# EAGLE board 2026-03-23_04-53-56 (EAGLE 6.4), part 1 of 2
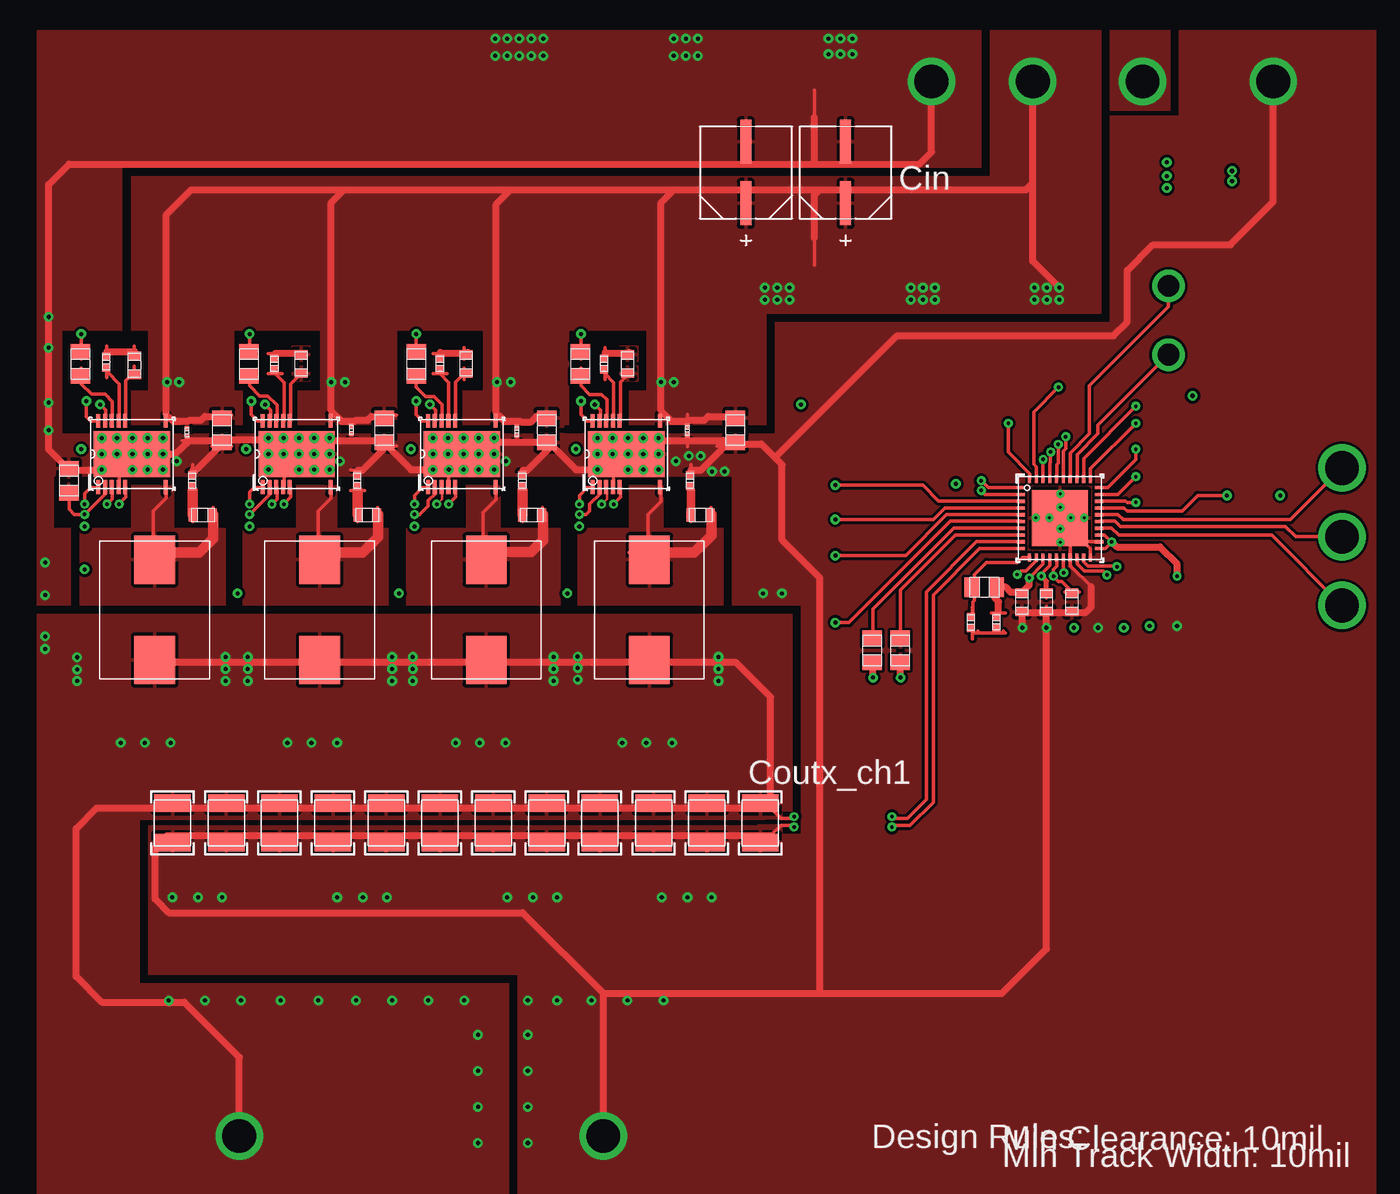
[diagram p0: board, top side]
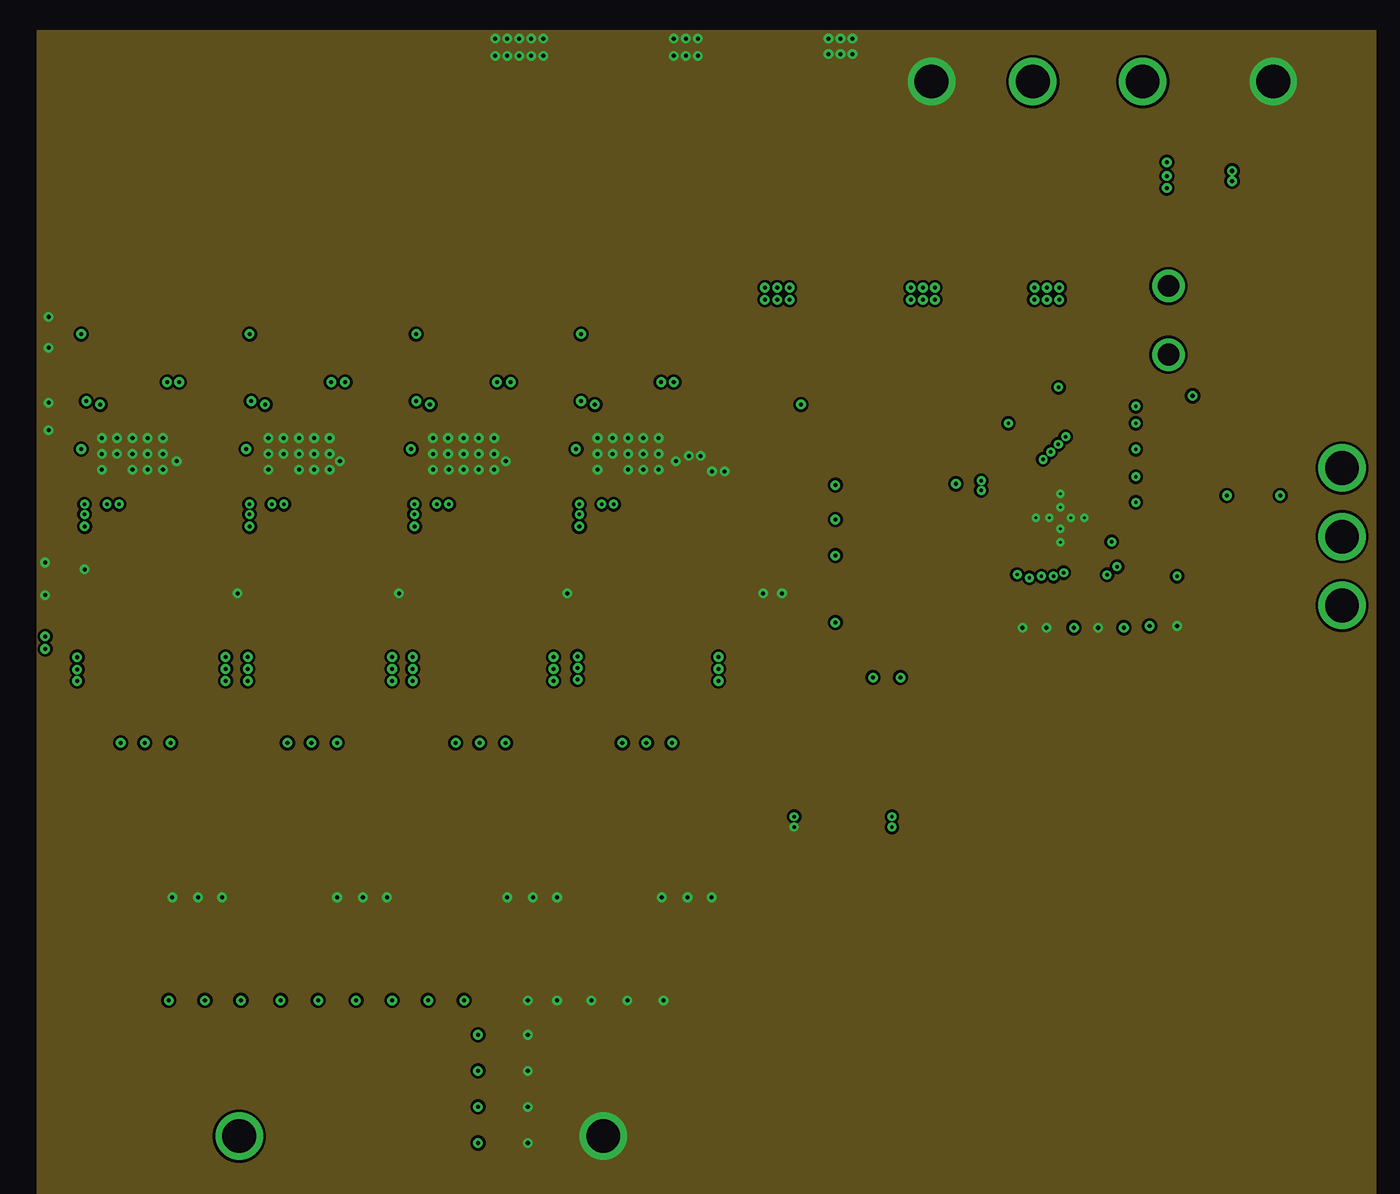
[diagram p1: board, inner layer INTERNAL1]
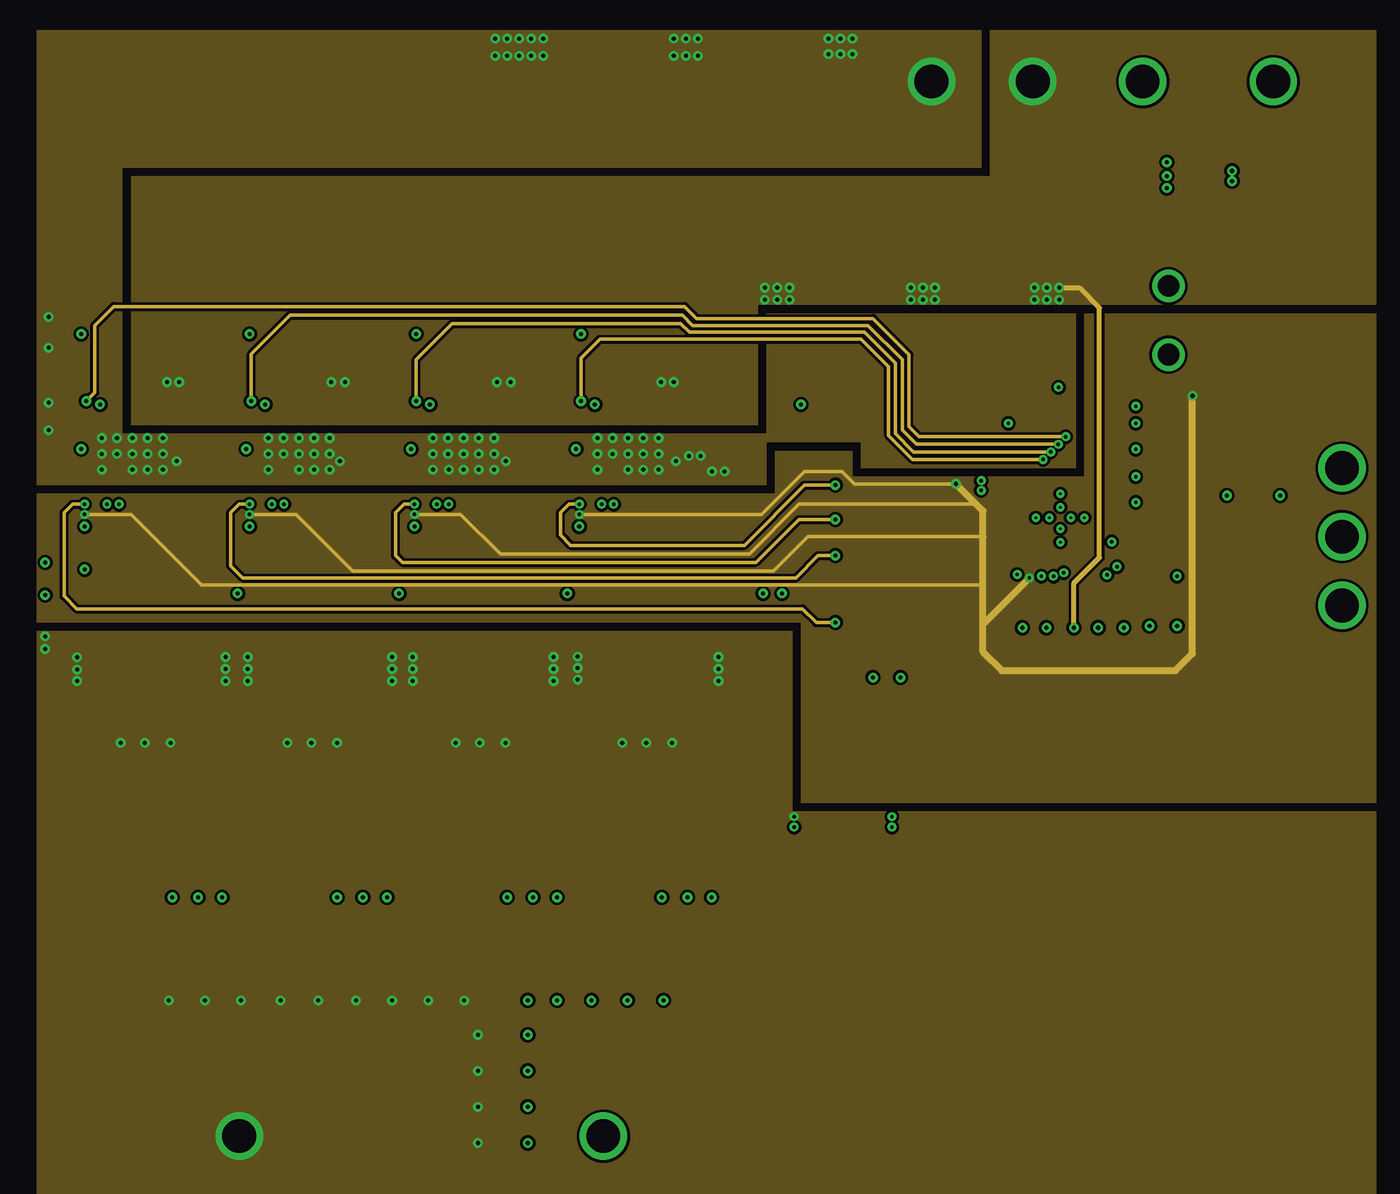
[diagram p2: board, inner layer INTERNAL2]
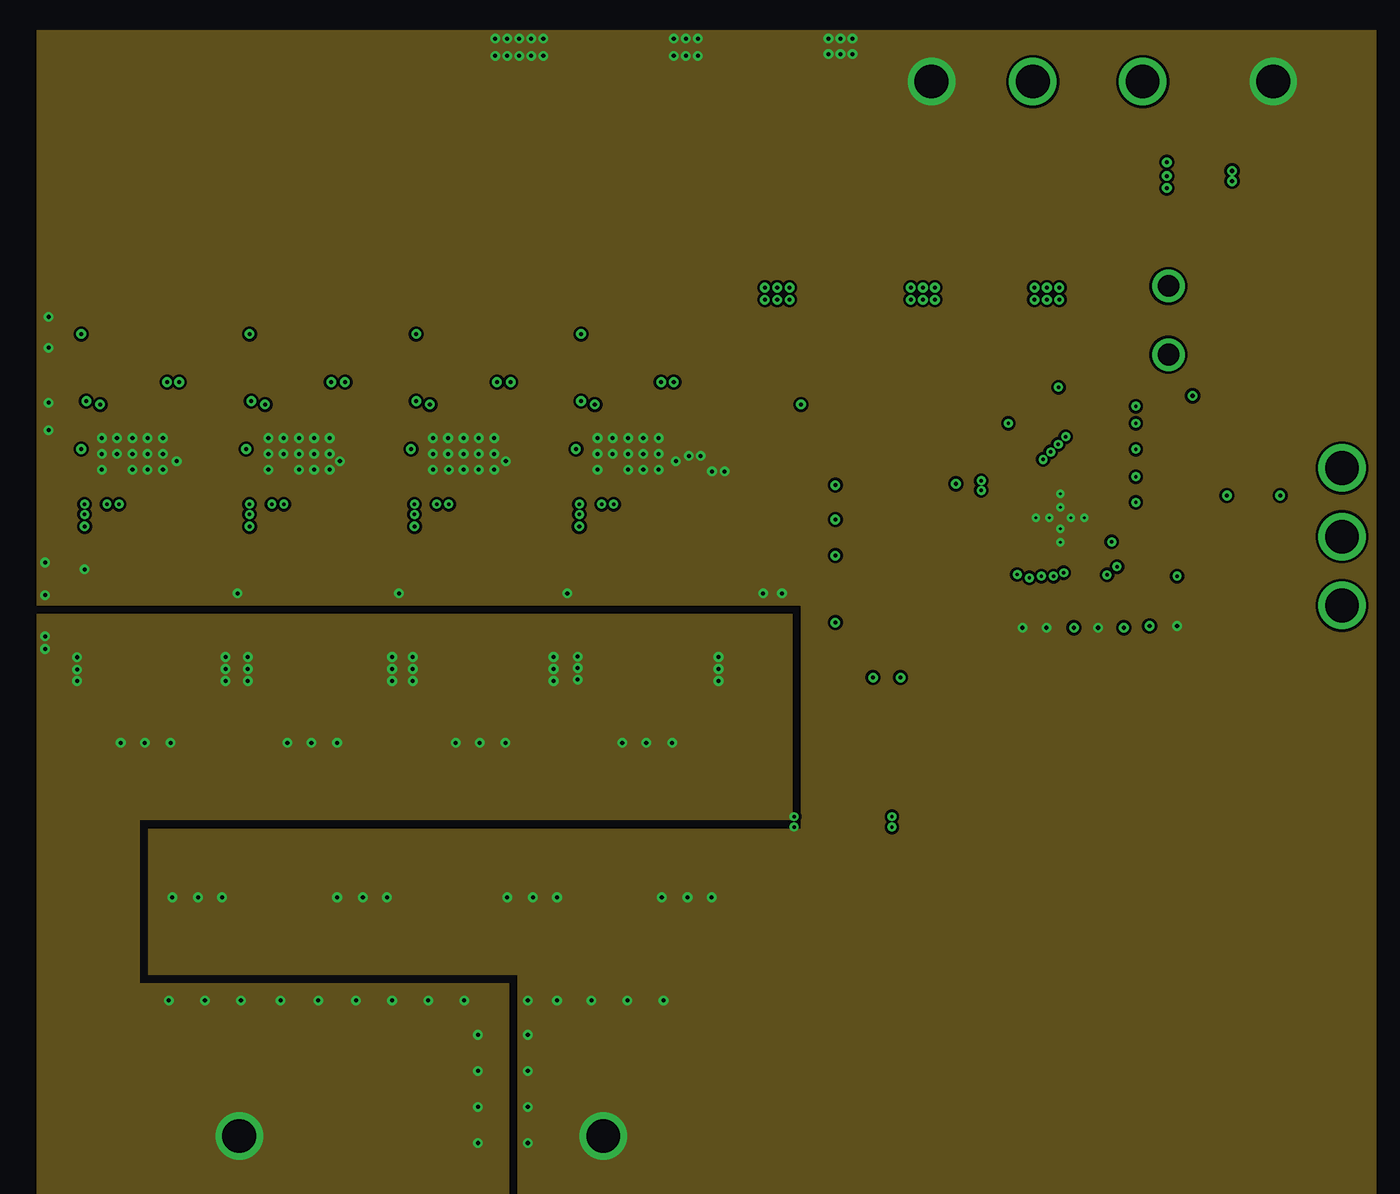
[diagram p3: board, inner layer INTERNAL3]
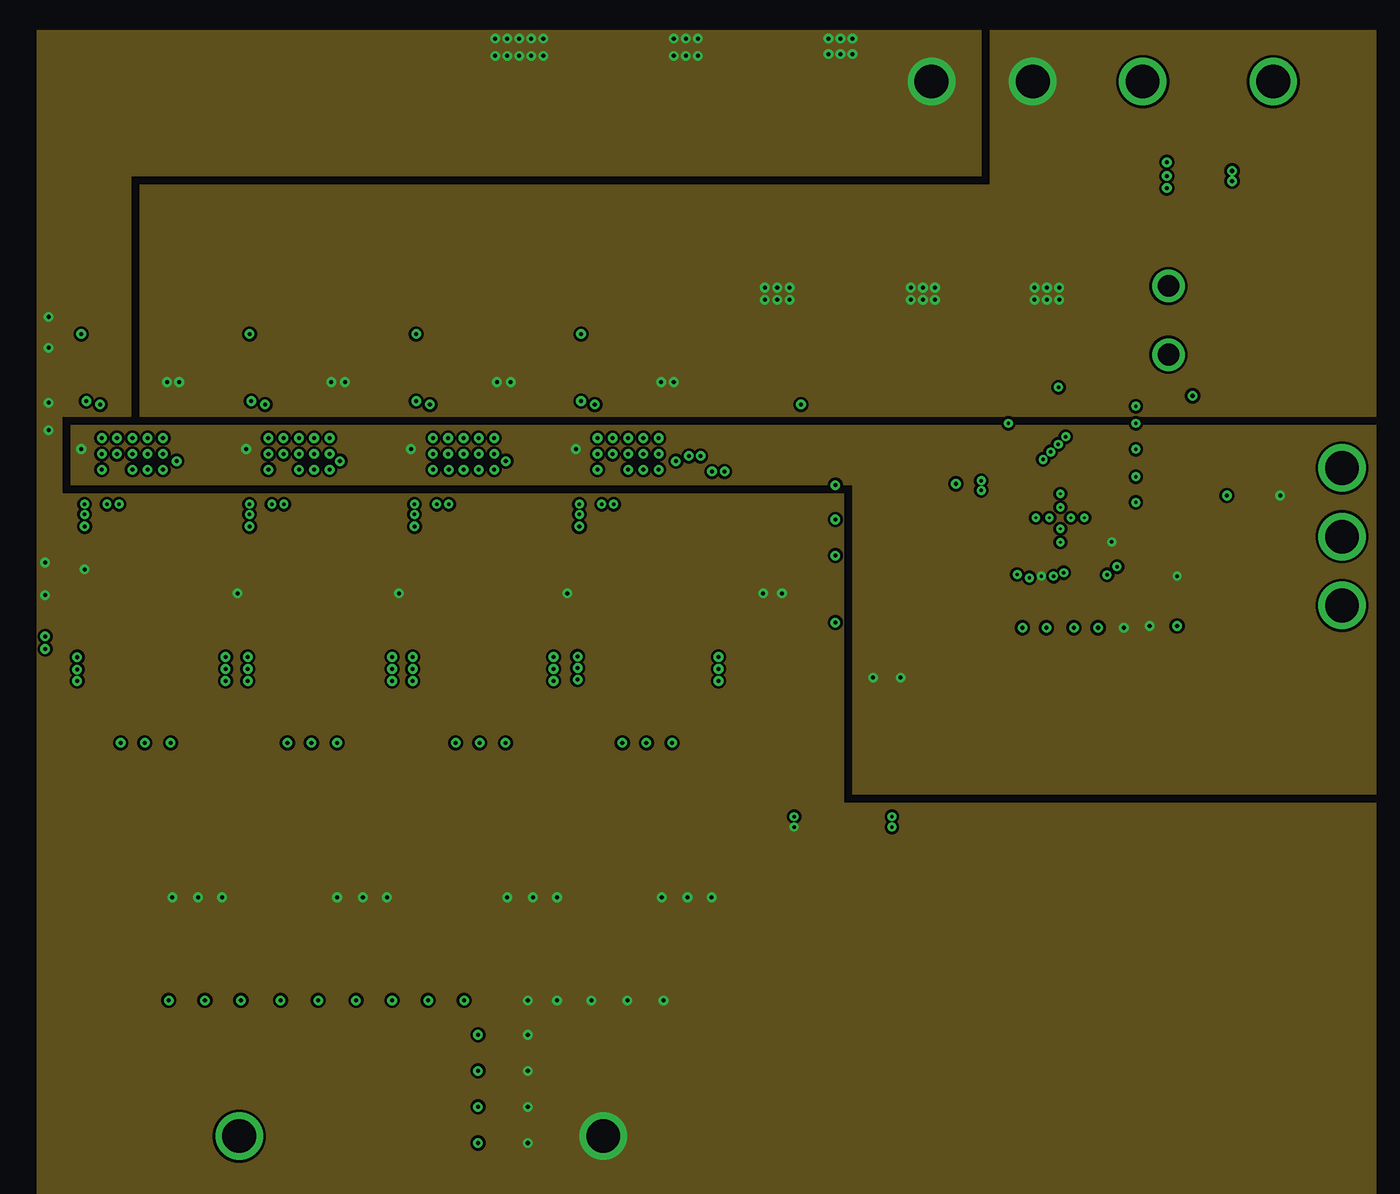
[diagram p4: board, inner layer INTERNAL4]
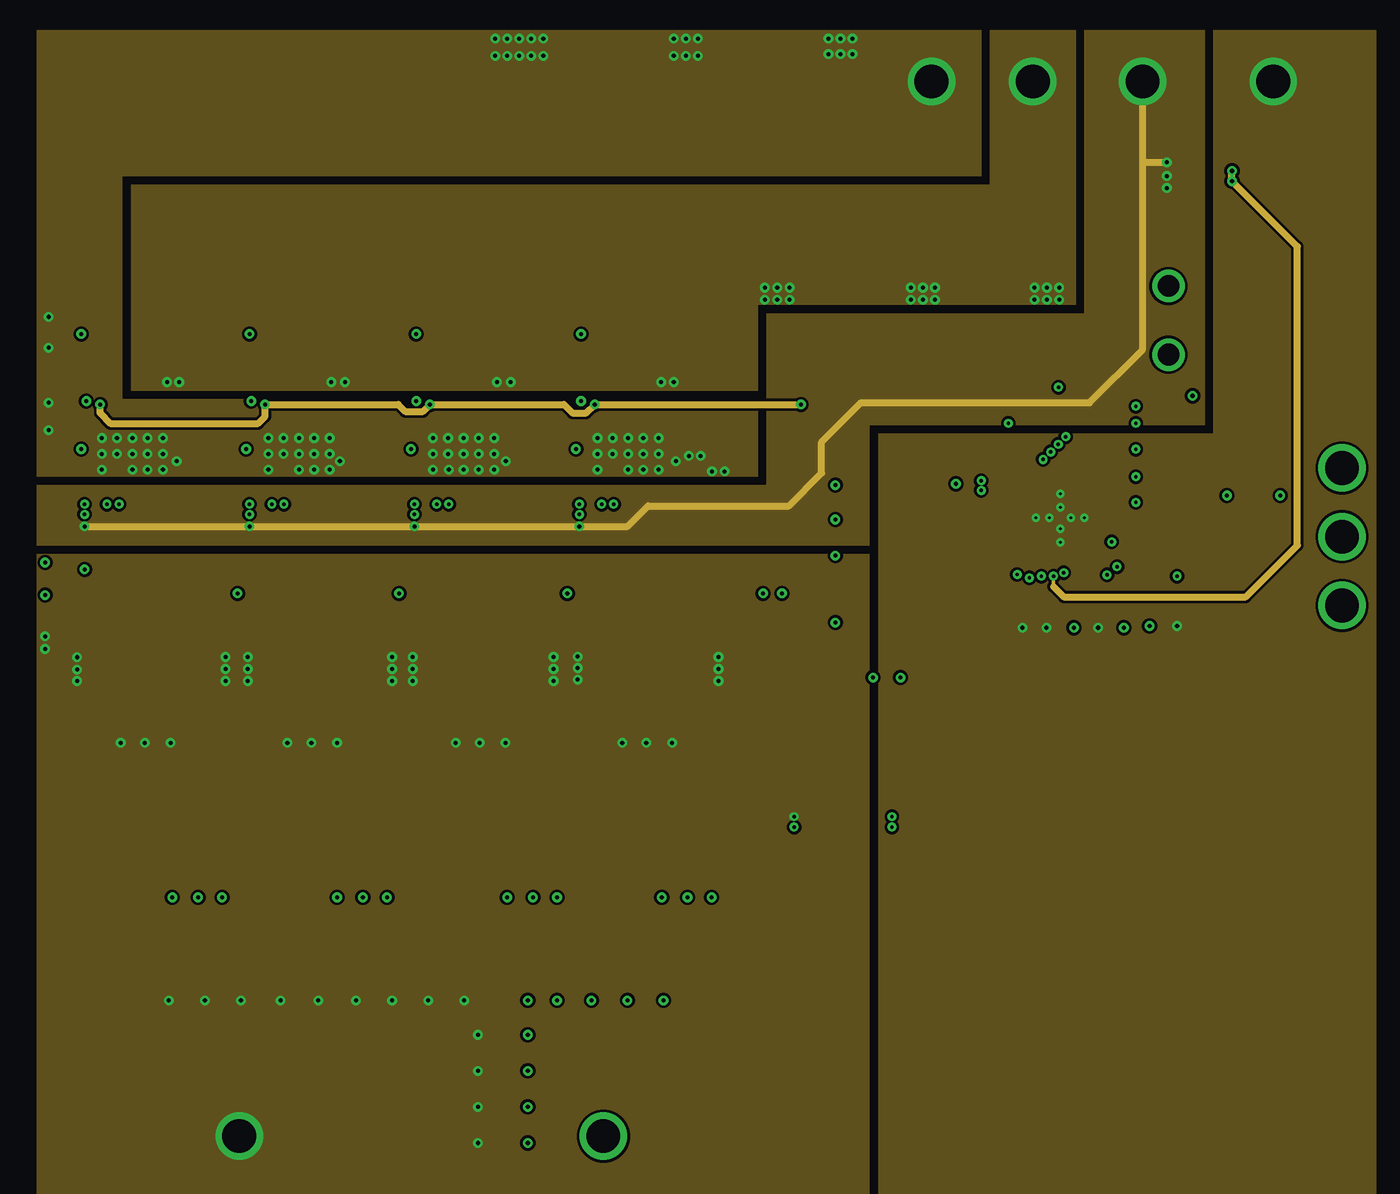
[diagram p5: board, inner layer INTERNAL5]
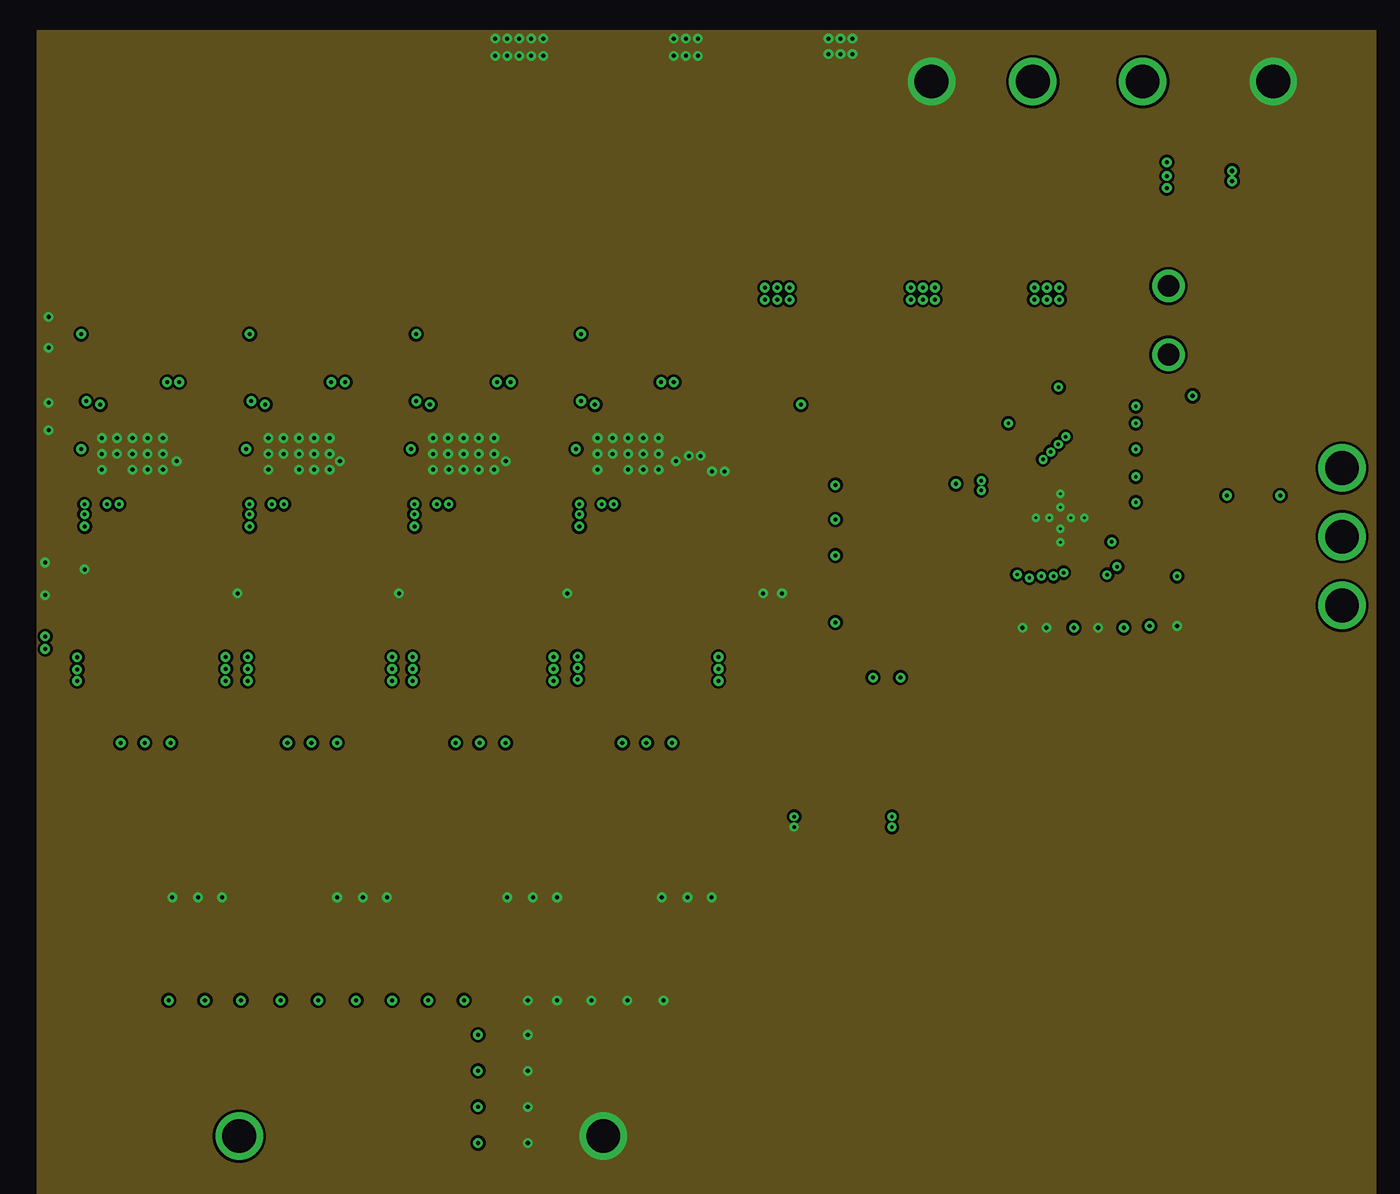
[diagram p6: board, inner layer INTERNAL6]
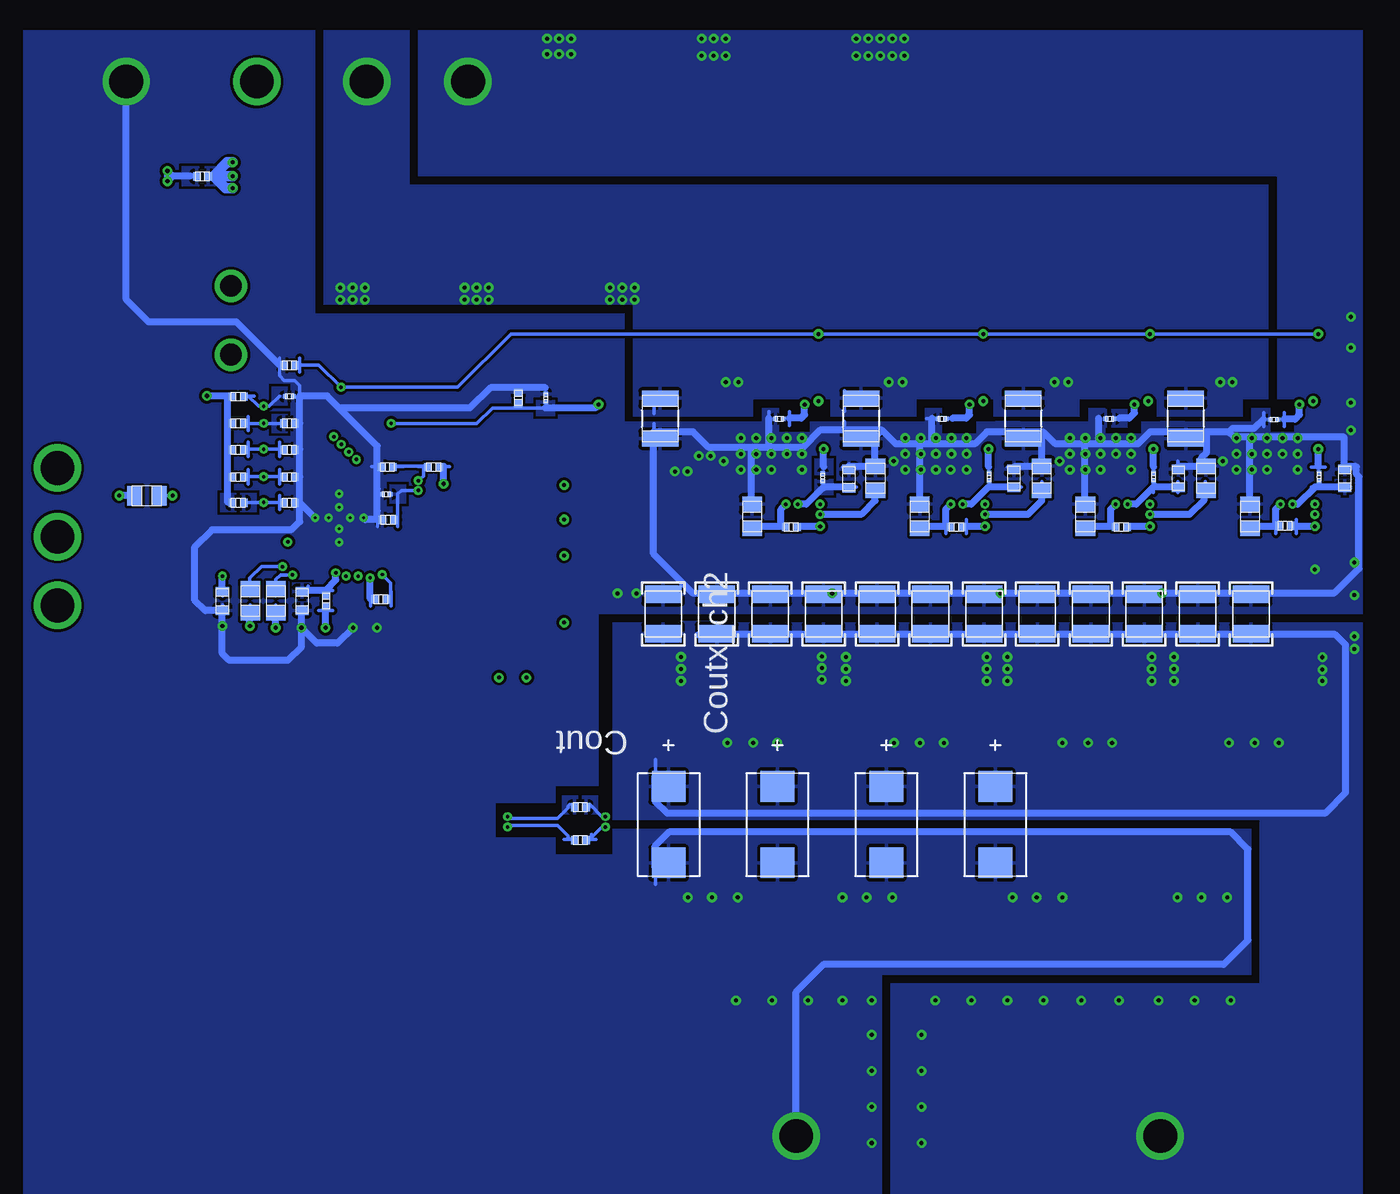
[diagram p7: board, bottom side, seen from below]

No outline drawn. Coordinates in mm, seen from the top.
Copper layers ((1*2)+(15*16)): TOP / INTERNAL1 / layer 15 / BOTTOM

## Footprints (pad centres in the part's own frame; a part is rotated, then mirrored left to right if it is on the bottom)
0603 = smd 0.66 x 0.965: 1 -0.699,0; 2 0.699,0
0402 = smd 0.559 x 0.61: 1 -0.419,0; 2 0.419,0
0805 = smd 1.118 x 1.448: 1 -0.902,0; 2 0.902,0
0201_033 = smd 0.356 x 0.33: 1 -0.292,0; 2 0.292,0
0201 = smd 0.356 x 0.33: 1 -0.292,0; 2 0.292,0
CAPSMT_62_C10 = smd 3.251 x 0.813: 1 -2.273,0; 2 2.273,0
1210_280 = smd 1.118 x 2.692: 1 -1.499,0; 2 1.499,0
7343-20 = smd 2.261 x 2.489: 1 -2.819,0; 2 2.819,0
1210_270 = smd 1.3 x 2.7: 1 -1.45,0; 2 1.45,0
TP-1502 = drill 0.813 pad 1.651 round: 1 0,0
WE-HCM_1088 = smd 3.56 x 3: 1 -3.71,0; 2 3.71,0
DQP0012A = smd 1 x 0.3: 1 -2.45,2.501; 2 -2.45,2.001; 3 -2.45,1.5; 4 -2.45,1; 5 -2.45,0.5; 6 -2.45,-2.501; 7 2.45,-2.501; 8 2.45,0.5; 9 2.45,1; 10 2.45,1.5; 11 2.45,2.001; 12 2.45,2.501 | smd 3.4 x 5.639: 13 0,0
TP-5012 = drill 0.813 pad 1.651 round: 1 0,0
RTA0040B = smd 0.6 x 0.23: 1 -2.9,2.25; 2 -2.9,1.75; 3 -2.9,1.25; 4 -2.9,0.75; 5 -2.9,0.25; 6 -2.9,-0.25; 7 -2.9,-0.75; 8 -2.9,-1.25; 9 -2.9,-1.75; 10 -2.9,-2.25; 21 2.9,-2.25; 22 2.9,-1.75; 23 2.9,-1.25; 24 2.9,-0.75; 25 2.9,-0.25; 26 2.9,0.25; 27 2.9,0.75; 28 2.9,1.25; 29 2.9,1.75; 30 2.9,2.25 | smd 0.23 x 0.6: 11 -2.25,-2.9; 12 -1.75,-2.9; 13 -1.25,-2.9; 14 -0.75,-2.9; 15 -0.25,-2.9; 16 0.25,-2.9; 17 0.75,-2.9; 18 1.25,-2.9; 19 1.75,-2.9; 20 2.25,-2.9; 31 2.25,2.9; 32 1.75,2.9; 33 1.25,2.9; 34 0.75,2.9; 35 0.25,2.9; 36 -0.25,2.9; 37 -0.75,2.9; 38 -1.25,2.9; 39 -1.75,2.9; 40 -2.25,2.9 | smd 4.15 x 4.15: 41 0,0

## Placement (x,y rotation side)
C3v3  [0603]  111,70.82 270 bottom
Cbp3  [0603]  101.35,70.71 270 top
Cbst1  [0603]  70.36,88.34 270 top
Cbst2  [0603]  58.42,88.34 270 top
Cbst3  [0603]  46.23,88.34 270 top
Cbst4  [0603]  33.91,88.24 270 top
Ccomp  [0402]  97.64,69.24 90 top
Ccomp2  [0805]  96.75,71.83 0 top
Cdd  [0603]  105.11,70.82 270 bottom
Cen1  [0603]  64.67,79.86 90 bottom
Cen2  [0603]  52.48,79.88 90 bottom
Cen3  [0603]  40.31,79.88 90 bottom
Cen4  [0603]  28.02,79.88 90 bottom
Chf1  [0201_033]  74.78,83.41 270 top
Chf2  [0201_033]  62.18,83.34 270 top
Chf3  [0201_033]  49.96,83.46 270 top
Chf4  [0201_033]  37.8,83.29 270 top
Cimon  [0201]  98.88,78.71 180 bottom
Cin_1  [CAPSMT_62_C10]  86.49,102.49 90 top
Cin_2  [CAPSMT_62_C10]  79.12,102.49 90 top
Cinx_ch1  [0805]  78.33,83.44 270 top
Cinx_ch2  [0805]  64.39,83.44 270 top
Cinx_ch3  [0805]  52.37,83.44 270 top
Cinx_ch4  [0805]  40.39,83.44 270 top
Cinx_ch5  [1210_280]  78.64,84.3 270 bottom
Cinx_ch6  [1210_280]  63.78,84.3 270 bottom
Cinx_ch7  [1210_280]  51.79,84.3 270 bottom
Cinx_ch8  [1210_280]  39.78,84.3 270 bottom
Cout_1  [7343-20]  78,54.28 270 bottom
Cout_2  [7343-20]  69.95,54.28 270 bottom
Cout_3  [7343-20]  61.9,54.28 270 bottom
Cout_4  [7343-20]  53.85,54.28 270 bottom
Coutx_ch1_1  [1210_270]  80.19,54.41 270 top
Coutx_ch1_2  [1210_270]  76.23,54.41 270 top
Coutx_ch1_3  [1210_270]  72.29,54.41 270 top
Coutx_ch1_4  [1210_270]  68.33,54.41 270 top
Coutx_ch1_5  [1210_270]  64.39,54.41 270 top
Coutx_ch1_6  [1210_270]  60.43,54.41 270 top
Coutx_ch1_7  [1210_270]  56.49,54.41 270 top
Coutx_ch1_8  [1210_270]  52.53,54.41 270 top
Coutx_ch1_9  [1210_270]  48.59,54.41 270 top
Coutx_ch1_10  [1210_270]  44.63,54.41 270 top
Coutx_ch1_11  [1210_270]  40.69,54.41 270 top
Coutx_ch1_12  [1210_270]  36.73,54.41 270 top
Coutx_ch2_1  [1210_270]  78.41,69.85 90 bottom
Coutx_ch2_2  [1210_270]  74.45,69.85 90 bottom
Coutx_ch2_3  [1210_270]  70.48,69.85 90 bottom
Coutx_ch2_4  [1210_270]  66.55,69.85 90 bottom
Coutx_ch2_5  [1210_270]  62.59,69.85 90 bottom
Coutx_ch2_6  [1210_270]  58.65,69.85 90 bottom
Coutx_ch2_7  [1210_270]  54.69,69.85 90 bottom
Coutx_ch2_8  [1210_270]  50.75,69.85 90 bottom
Coutx_ch2_9  [1210_270]  46.79,69.85 90 bottom
Coutx_ch2_10  [1210_270]  42.85,69.85 90 bottom
Coutx_ch2_11  [1210_270]  38.89,69.85 90 bottom
Coutx_ch2_12  [1210_270]  34.95,69.85 90 bottom
Cref  [0603]  99.52,70.71 270 top
Cref1  [0805]  62.71,79.88 90 bottom
Cref2  [0805]  50.42,79.88 90 bottom
Cref3  [0805]  38.28,79.88 90 bottom
Cref4  [0805]  29.06,79.71 90 top
Csnub1  [0603]  75.77,77.17 180 top
Csnub2  [0603]  63.3,77.17 180 top
Csnub3  [0603]  51.13,77.17 180 top
Csnub4  [0603]  38.96,77.17 180 top
Ctao1  [0201]  69.82,84.28 180 bottom
Ctao2  [0201]  57.78,84.28 180 bottom
Ctao3  [0201]  45.39,84.28 180 bottom
Ctao4  [0201]  33.25,84.23 180 bottom
Ctsen  [0201]  87.07,85.83 90 bottom
Cv5  [0603]  103.23,70.71 270 top
Cvdd1  [0805]  71.83,77.06 90 bottom
Cvdd2  [0805]  59.44,77.06 90 bottom
Cvdd3  [0805]  47.19,77.06 90 bottom
Cvdd4  [0805]  35.03,77.06 90 bottom
GND  [TP-1502]  92.84,109.17 0 top
GND1  [TP-1502]  68.53,31.19 0 top
GND2  [TP-1502]  118.08,109.17 0 top
L1  [WE-HCM_1088]  71.98,70.15 270 top
L2  [WE-HCM_1088]  59.92,70.15 270 top
L3  [WE-HCM_1088]  47.6,70.15 270 top
L4  [WE-HCM_1088]  35.41,70.15 270 top
M1  [DQP0012A]  70.28,81.69 90 top
M2  [DQP0012A]  58.12,81.69 90 top
M3  [DQP0012A]  45.9,81.69 90 top
M4  [DQP0012A]  33.73,81.69 90 top
NC3  [TP-5012]  110.34,88.98 0 top
NC4  [TP-5012]  110.34,94.03 0 top
Raddr  [0402]  109.83,78.08 0 bottom
Rbst1  [0402]  68.63,88.34 270 top
Rbst2  [0402]  56.49,88.34 270 top
Rbst3  [0402]  44.25,88.34 270 top
Rbst4  [0402]  31.83,88.47 270 top
Rcomp  [0402]  95.76,69.22 90 top
Rdd  [0402]  103.33,70.82 270 bottom
Ren1  [0201]  66.6,79.93 270 bottom
Ren2  [0201]  54.31,79.98 270 bottom
Ren3  [0201]  42.14,79.98 270 bottom
Ren4  [0201]  29.92,79.98 270 bottom
Rf  [0201]  106.05,85.93 0 bottom
Rfccm1  [0805]  66.88,88.34 270 top
Rfccm2  [0805]  54.74,88.34 270 top
Rfccm3  [0805]  42.37,88.34 270 top
Rfccm4  [0805]  29.92,88.34 270 top
Rimax  [0402]  109.83,85.93 0 bottom
Rimon  [0402]  98.76,76.81 180 bottom
Risum  [0402]  99.29,70.94 0 bottom
Rmode  [0402]  109.83,79.98 0 bottom
Rnc1  [0805]  90.53,67.16 90 top
Rnc2  [0805]  88.47,67.16 90 top
Rnvm  [0402]  106.05,88.24 180 bottom
Rocpr  [0402]  98.81,80.72 180 bottom
Rosr  [0402]  106.05,81.99 0 bottom
Rramp  [0402]  95.38,80.72 180 bottom
Rslew  [0402]  106.05,79.98 0 bottom
Rsn  [0402]  84.53,53.14 180 bottom
Rsnub1  [0402]  74.98,79.71 90 top
Rsnub2  [0402]  62.59,79.71 90 top
Rsnub3  [0402]  50.37,79.71 90 top
Rsnub4  [0402]  38.18,79.71 90 top
Rsp  [0402]  84.53,55.58 180 bottom
Rtrise  [0402]  106.05,78.08 0 bottom
Rtsen  [0402]  89.13,85.83 90 bottom
Rusr  [0402]  109.83,81.99 0 bottom
Rv5  [0402]  112.47,102.21 180 bottom
Rvbootb  [0402]  106.05,83.95 0 bottom
Rvboott  [0402]  109.83,83.95 0 bottom
Rvdd1  [0402]  68.94,76.28 0 bottom
Rvdd2  [0402]  56.72,76.28 0 bottom
Rvdd3  [0402]  44.53,76.28 0 bottom
Rvdd4  [0402]  32.44,76.38 0 bottom
Rvr_fault  [0805]  116.59,78.59 0 bottom
Rvr_hot  [0805]  108.92,70.82 90 bottom
Rvr_rdy  [0805]  107.04,70.82 90 bottom
U1  [RTA0040B]  102.34,76.94 0 top
V5  [TP-1502]  108.43,109.17 0 top
Valert  [TP-1502]  123.16,75.54 0 top
VIN  [TP-1502]  100.28,109.17 0 top
VOUT  [TP-1502]  41.61,31.19 0 top
Vscl  [TP-1502]  123.16,70.48 0 top
Vsda  [TP-1502]  123.16,80.64 0 top

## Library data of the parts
C3v3 = ultra-librarian; RefDes: C3v3; Type: C0603C105Z8VACTU
Cbp3 = ultra-librarian; RefDes: Cbp3; Type: C0603C105Z8VACTU
Cbst1 = ultra-librarian; RefDes: Cbst1; Type: EMK107B7104KA-T
Cbst2 = ultra-librarian; RefDes: Cbst2; Type: EMK107B7104KA-T
Cbst3 = ultra-librarian; RefDes: Cbst3; Type: EMK107B7104KA-T
Cbst4 = ultra-librarian; RefDes: Cbst4; Type: EMK107B7104KA-T
Ccomp = ultra-librarian; RefDes: Ccomp; Type: GRM1555C1H102JA01J
Ccomp2 = ultra-librarian; RefDes: Ccomp2; Type: CL21C220JBANNNC
Cdd = ultra-librarian; RefDes: Cdd; Type: C1608X5R1E105K080AC
Cen1 = ultra-librarian; RefDes: Cen1; Type: CC0603JRNPO8BN102
Cen2 = ultra-librarian; RefDes: Cen2; Type: CC0603JRNPO8BN102
Cen3 = ultra-librarian; RefDes: Cen3; Type: CC0603JRNPO8BN102
Cen4 = ultra-librarian; RefDes: Cen4; Type: CC0603JRNPO8BN102
Chf1 = ultra-librarian; RefDes: Chf1; Type: CGA1A2X7R1E332K030BA
Chf2 = ultra-librarian; RefDes: Chf2; Type: CGA1A2X7R1E332K030BA
Chf3 = ultra-librarian; RefDes: Chf3; Type: CGA1A2X7R1E332K030BA
Chf4 = ultra-librarian; RefDes: Chf4; Type: CGA1A2X7R1E332K030BA
Cimon = ultra-librarian; RefDes: Cimon; Type: GRM033R71A222KA01D
Cin_1 Cin_2 Cout_1-Cout_4 Coutx_ch1_1-Coutx_ch1_12 Coutx_ch2_1-Coutx_ch2_12 M1-M4 = ultra-librarian
Cinx_ch1 = ultra-librarian; RefDes: Cinx_ch1; Type: MSASE21GBB5226MTNA01
Cinx_ch2 = ultra-librarian; RefDes: Cinx_ch2; Type: MSASE21GBB5226MTNA01
Cinx_ch3 = ultra-librarian; RefDes: Cinx_ch3; Type: MSASE21GBB5226MTNA01
Cinx_ch4 = ultra-librarian; RefDes: Cinx_ch4; Type: MSASE21GBB5226MTNA01
Cinx_ch5 = ultra-librarian; RefDes: Cinx_ch5; Type: GRM32ER61C476KE15L
Cinx_ch6 = ultra-librarian; RefDes: Cinx_ch6; Type: GRM32ER61C476KE15L
Cinx_ch7 = ultra-librarian; RefDes: Cinx_ch7; Type: GRM32ER61C476KE15L
Cinx_ch8 = ultra-librarian; RefDes: Cinx_ch8; Type: GRM32ER61C476KE15L
Cref = ultra-librarian; RefDes: Cref; Type: C0603C334K8RACTU
Cref1 = ultra-librarian; RefDes: Cref1; Type: 08053C104KAT2A
Cref2 = ultra-librarian; RefDes: Cref2; Type: 08053C104KAT2A
Cref3 = ultra-librarian; RefDes: Cref3; Type: 08053C104KAT2A
Cref4 = ultra-librarian; RefDes: Cref4; Type: 08053C104KAT2A
Csnub1 = ultra-librarian; RefDes: Csnub1; Type: CC0603JRNPO8BN102
Csnub2 = ultra-librarian; RefDes: Csnub2; Type: CC0603JRNPO8BN102
Csnub3 = ultra-librarian; RefDes: Csnub3; Type: CC0603JRNPO8BN102
Csnub4 = ultra-librarian; RefDes: Csnub4; Type: CC0603JRNPO8BN102
Ctao1 = ultra-librarian; RefDes: Ctao1; Type: GRM033R71C102KA01D
Ctao2 = ultra-librarian; RefDes: Ctao2; Type: GRM033R71C102KA01D
Ctao3 = ultra-librarian; RefDes: Ctao3; Type: GRM033R71C102KA01D
Ctao4 = ultra-librarian; RefDes: Ctao4; Type: GRM033R71C102KA01D
Ctsen = ultra-librarian; RefDes: Ctsen; Type: GRM033R71C102KA01D
Cv5 = ultra-librarian; RefDes: Cv5; Type: C1608X5R1C475K080AC
Cvdd1 = ultra-librarian; RefDes: Cvdd1; Type: EMK212BJ225KG-T
Cvdd2 = ultra-librarian; RefDes: Cvdd2; Type: EMK212BJ225KG-T
Cvdd3 = ultra-librarian; RefDes: Cvdd3; Type: EMK212BJ225KG-T
Cvdd4 = ultra-librarian; RefDes: Cvdd4; Type: EMK212BJ225KG-T
GND = ultra-librarian; RefDes: GND; Type: TP-1502
GND1 = ultra-librarian; RefDes: GND1; Type: TP-1502
GND2 = ultra-librarian; RefDes: GND2; Type: TP-1502
L1 = ultra-librarian; RefDes: L1; Type: 7443082022
L2 = ultra-librarian; RefDes: L2; Type: 7443082022
L3 = ultra-librarian; RefDes: L3; Type: 7443082022
L4 = ultra-librarian; RefDes: L4; Type: 7443082022
NC3 = ultra-librarian; RefDes: NC3; Type: TP-5012
NC4 = ultra-librarian; RefDes: NC4; Type: TP-5012
Raddr = ultra-librarian; RefDes: Raddr; Type: CRCW040216K5FKED
Rbst1 = ultra-librarian; RefDes: Rbst1; Type: CRCW04021R00FKED
Rbst2 = ultra-librarian; RefDes: Rbst2; Type: CRCW04021R00FKED
Rbst3 = ultra-librarian; RefDes: Rbst3; Type: CRCW04021R00FKED
Rbst4 = ultra-librarian; RefDes: Rbst4; Type: CRCW04021R00FKED
Rcomp = ultra-librarian; RefDes: Rcomp; Type: CRCW04023K83FKED
Rdd = ultra-librarian; RefDes: Rdd; Type: CRCW04021R00FKED
Ren1 = ultra-librarian; RefDes: Ren1; Type: RC0201FR-0710KL
Ren2 = ultra-librarian; RefDes: Ren2; Type: RC0201FR-0710KL
Ren3 = ultra-librarian; RefDes: Ren3; Type: RC0201FR-0710KL
Ren4 = ultra-librarian; RefDes: Ren4; Type: RC0201FR-0710KL
Rf = ultra-librarian; RefDes: Rf; Type: RC0201FR-0723K7L
Rfccm1 = ultra-librarian; RefDes: Rfccm1; Type: ERJ-6ENF2372V
Rfccm2 = ultra-librarian; RefDes: Rfccm2; Type: ERJ-6ENF2372V
Rfccm3 = ultra-librarian; RefDes: Rfccm3; Type: ERJ-6ENF2372V
Rfccm4 = ultra-librarian; RefDes: Rfccm4; Type: ERJ-6ENF2372V
Rimax = ultra-librarian; RefDes: Rimax; Type: CRCW040226K1FKED
Rimon = ultra-librarian; RefDes: Rimon; Type: CRCW040249K9FKED
Risum = ultra-librarian; RefDes: Risum; Type: CRCW04022K55FKED
Rmode = ultra-librarian; RefDes: Rmode; Type: CRCW040216K5FKED
Rnc1 = ultra-librarian; RefDes: Rnc1; Type: ERJ-6ENF2002V
Rnc2 = ultra-librarian; RefDes: Rnc2; Type: ERJ-6ENF2002V
Rnvm = ultra-librarian; RefDes: Rnvm; Type: CRCW040220K0FKED
Rocpr = ultra-librarian; RefDes: Rocpr; Type: CRCW040220K0FKED
Rosr = ultra-librarian; RefDes: Rosr; Type: CRCW0402150KFKED
Rramp = ultra-librarian; RefDes: Rramp; Type: CRCW04024K32FKED
Rslew = ultra-librarian; RefDes: Rslew; Type: CRCW040224K3FKED
Rsn = ultra-librarian; RefDes: Rsn; Type: CRCW04021R00FKED
Rsnub1 = ultra-librarian; RefDes: Rsnub1; Type: CRCW04021R00FKED
Rsnub2 = ultra-librarian; RefDes: Rsnub2; Type: CRCW04021R00FKED
Rsnub3 = ultra-librarian; RefDes: Rsnub3; Type: CRCW04021R00FKED
Rsnub4 = ultra-librarian; RefDes: Rsnub4; Type: CRCW04021R00FKED
Rsp = ultra-librarian; RefDes: Rsp; Type: CRCW04021R00FKED
Rtrise = ultra-librarian; RefDes: Rtrise; Type: CRCW040224K3FKED
Rtsen = ultra-librarian; RefDes: Rtsen; Type: CRCW0402121KFKED
Rusr = ultra-librarian; RefDes: Rusr; Type: CRCW04029K31FKED
Rv5 = ultra-librarian; RefDes: Rv5; Type: CRCW04021R00FKED
Rvbootb = ultra-librarian; RefDes: Rvbootb; Type: CRCW040239K2FKED
Rvboott = ultra-librarian; RefDes: Rvboott; Type: CRCW040226K7FKED
Rvdd1 = ultra-librarian; RefDes: Rvdd1; Type: CRCW04021R00FKED
Rvdd2 = ultra-librarian; RefDes: Rvdd2; Type: CRCW04021R00FKED
Rvdd3 = ultra-librarian; RefDes: Rvdd3; Type: CRCW04021R00FKED
Rvdd4 = ultra-librarian; RefDes: Rvdd4; Type: CRCW04021R00FKED
Rvr_fault = ultra-librarian; RefDes: Rvr_fault; Type: CRCW08051R00FKEA
Rvr_hot = ultra-librarian; RefDes: Rvr_hot; Type: CRCW08051R00FKEA
Rvr_rdy = ultra-librarian; RefDes: Rvr_rdy; Type: CRCW08051R00FKEA
U1 = ultra-librarian; RefDes: U1; Type: TPS53647RTAR
V5 = ultra-librarian; RefDes: V5; Type: TP-1502
Valert = ultra-librarian; RefDes: Valert; Type: TP-1502
VIN = ultra-librarian; RefDes: VIN; Type: TP-1502
VOUT = ultra-librarian; RefDes: VOUT; Type: TP-1502
Vscl = ultra-librarian; RefDes: Vscl; Type: TP-1502
Vsda = ultra-librarian; RefDes: Vsda; Type: TP-1502

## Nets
0: C3v3.2 Cbp3.2 Cdd.2 Cen1.2 Cen2.2 Cen3.2 Cen4.2 Chf1.2 Chf2.2 Chf3.2 Chf4.2 Cimon.2 Cin_1.2 Cin_2.2 Cinx_ch1.2 Cinx_ch2.2 Cinx_ch3.2 Cinx_ch4.2 Cinx_ch5.2 Cinx_ch6.2 Cinx_ch7.2 Cinx_ch8.2 Cout_1.2 Cout_2.2 Cout_3.2 Cout_4.2 Coutx_ch1_1.2 Coutx_ch1_2.2 Coutx_ch1_3.2 Coutx_ch1_4.2 Coutx_ch1_5.2 Coutx_ch1_6.2 Coutx_ch1_7.2 Coutx_ch1_8.2 Coutx_ch1_9.2 Coutx_ch1_10.2 Coutx_ch1_11.2 Coutx_ch1_12.2 Coutx_ch2_1.2 Coutx_ch2_2.2 Coutx_ch2_3.2 Coutx_ch2_4.2 Coutx_ch2_5.2 Coutx_ch2_6.2 Coutx_ch2_7.2 Coutx_ch2_8.2 Coutx_ch2_9.2 Coutx_ch2_10.2 Coutx_ch2_11.2 Coutx_ch2_12.2 Cref1.2 Cref2.2 Cref3.2 Cref4.2 Cref.2 Ctao1.2 Ctao2.2 Ctao3.2 Ctao4.2 Ctsen.2 Cv5.2 Cvdd1.2 Cvdd2.2 Cvdd3.2 Cvdd4.2 GND1.1 GND2.1 GND.1 M1.4 M1.13 M2.4 M2.13 M3.4 M3.13 M4.4 M4.13 Rf.2 Rimon.2 Rnvm.2 Rocpr.2 Rosr.2 Rslew.2 Rsn.1 Rsnub1.2 Rsnub2.2 Rsnub3.2 Rsnub4.2 Rtrise.2 Rtsen.2 Rvbootb.2 U1.17 U1.20 U1.22 U1.41
1: Chf1.1 Chf2.1 Chf3.1 Chf4.1 Cin_1.1 Cin_2.1 Cinx_ch1.1 Cinx_ch2.1 Cinx_ch3.1 Cinx_ch4.1 Cinx_ch5.1 Cinx_ch6.1 Cinx_ch7.1 Cinx_ch8.1 M1.7 M2.7 M3.7 M4.7 Rdd.2 VIN.1
2: Rocpr.1 Rramp.2 U1.1
5: Rf.1 Rimax.2 U1.32
6: Rvbootb.1 Rvboott.2 U1.31
7: Rosr.1 Rusr.2 U1.30
9: Rmode.2 Rslew.1 U1.29
10: Raddr.2 Rtrise.1 U1.28
22: Cdd.1 Rdd.1 U1.16
23: Cv5.1 Rv5.2 U1.15
24: Rv5.1 Rvdd1.2 Rvdd2.2 Rvdd3.2 Rvdd4.2 V5.1
30: Ccomp2.1 Rcomp.2 U1.11
31: Cimon.1 Rimon.1 U1.2
34: Cvdd4.1 M4.5 Rvdd4.1
35: Cvdd3.1 M3.5 Rvdd3.1
36: Cvdd2.1 M2.5 Rvdd2.1
37: Cvdd1.1 M1.5 Rvdd1.1
38: Cen3.1 M3.3 Ren3.2
39: Cen2.1 M2.3 M3.10 Ren2.2 Rfccm3.2
40: Cbst3.2 Cen4.1 M3.8 M4.3 Ren4.2
41: Cen1.1 M1.3 Ren1.2
45: Ctao1.1 Ctao2.1 Ctao3.1 Ctao4.1 Ctsen.1 M1.11 M2.11 M3.11 M4.11 NC3.1 NC4.1 Rtsen.1 U1.33 U1.34 U1.40
56: Ccomp2.2 Ccomp.2 Cref1.1 Cref2.1 Cref3.1 Cref4.1 Cref.1 M1.2 M2.2 M3.2 M4.2 Raddr.1 Rimax.1 Risum.1 Rmode.1 Rramp.1 Rusr.1 Rvboott.1 U1.13
62: Cout_1.1 Cout_2.1 Cout_3.1 Cout_4.1 Coutx_ch1_1.1 Coutx_ch1_2.1 Coutx_ch1_3.1 Coutx_ch1_4.1 Coutx_ch1_5.1 Coutx_ch1_6.1 Coutx_ch1_7.1 Coutx_ch1_8.1 Coutx_ch1_9.1 Coutx_ch1_10.1 Coutx_ch1_11.1 Coutx_ch1_12.1 Coutx_ch2_1.1 Coutx_ch2_2.1 Coutx_ch2_3.1 Coutx_ch2_4.1 Coutx_ch2_5.1 Coutx_ch2_6.1 Coutx_ch2_7.1 Coutx_ch2_8.1 Coutx_ch2_9.1 Coutx_ch2_10.1 Coutx_ch2_11.1 Coutx_ch2_12.1 L1.2 L2.2 L3.2 L4.2 Rsp.1 VOUT.1
65: Ccomp.1 Rcomp.1
69: C3v3.1 Cbp3.1 Cbst4.2 M4.8 M4.10 Ren1.1 Ren2.1 Ren3.1 Ren4.1 Rfccm4.2 Rnc1.1 Rnc2.1 Rvr_fault.1 Rvr_hot.1 Rvr_rdy.1 U1.14 U1.21 U1.23
74: Csnub3.2 Rsnub3.1
75: Csnub2.2 Rsnub2.1
76: Csnub4.2 Rsnub4.1
77: Csnub1.2 Rsnub1.1
78: Cbst3.1 Rbst3.1
79: Cbst2.1 Rbst2.1
80: Cbst4.1 Rbst4.1
81: Cbst1.1 Rbst1.1
84: Csnub1.1 L1.1 M1.6
85: Csnub2.1 L2.1 M2.6
86: Csnub3.1 L3.1 M3.6
87: Csnub4.1 L4.1 M4.6
95: Cbst2.2 M2.8
107: Rvr_rdy.2 U1.18
108: Rvr_fault.2 U1.27
109: Risum.2 U1.12
110: Rfccm1.1 Rfccm2.1 Rfccm3.1 Rfccm4.1 Rnvm.1 U1.39
115: Rsp.2 U1.9
116: Rsn.2 U1.10
118: Rvr_hot.2 U1.19
123: M4.12 U1.35
124: M3.12 U1.36
125: M2.12 U1.37
126: M1.12 U1.38
127: U1.26 Vsda.1
128: U1.24 Vscl.1
129: U1.25 Valert.1
134: M4.1 U1.6
135: M3.1 U1.5
136: M2.1 U1.4
137: M1.1 U1.3
140: M2.9 Rbst2.2
144: M1.9 Rbst1.2
145: Cbst1.2 M1.8
146: M1.10 Rfccm1.2
148: M2.10 Rfccm2.2
150: M4.9 Rbst4.2
155: M3.9 Rbst3.2
158: Rnc2.2 U1.7
159: Rnc1.2 U1.8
